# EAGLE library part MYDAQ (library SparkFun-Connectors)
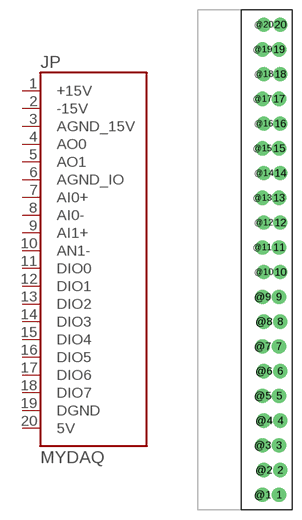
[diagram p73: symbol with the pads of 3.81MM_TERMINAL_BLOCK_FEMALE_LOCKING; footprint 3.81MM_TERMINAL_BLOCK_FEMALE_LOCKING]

Designator prefix JP

## MYDAQ  [3.81MM_TERMINAL_BLOCK_FEMALE_LOCKING]
1  +15V  pwr
2  -15V  pwr
3  AGND_15V  pwr
4  AO0  out
5  AO1  out
6  AGND_IO  pwr
7  AI0+  in
8  AI0-  in
9  AI1+  in
10  AN1-  in
11  DIO0
12  DIO1
13  DIO2
14  DIO3
15  DIO4
16  DIO5
17  DIO6
18  DIO7
19  DGND  pwr
20  5V  pwr

## Footprint 3.81MM_TERMINAL_BLOCK_FEMALE_LOCKING (pad centres in mm)
drill 1.2 pad 2.184: 1 4.521,-36.194; 2 4.724,-32.384; 3 4.521,-28.574; 4 4.724,-24.764; 5 4.521,-20.954; 6 4.724,-17.144; 7 4.521,-13.334; 8 4.724,-9.524; 9 4.521,-5.714; 10 4.724,-1.904; 11 4.521,1.906; 12 4.724,5.716; 13 4.521,9.526; 14 4.724,13.336; 15 4.521,17.146; 16 4.724,20.956; 17 4.521,24.766; 18 4.724,28.576; 19 4.521,32.386; 20 4.724,36.196; @1 1.981,-36.194; @2 2.184,-32.384; @3 1.981,-28.574; @4 2.184,-24.764; @5 1.981,-20.954; @6 2.184,-17.144; @7 1.981,-13.334; @8 2.184,-9.524; @9 1.981,-5.714; @10 2.184,-1.904; @11 1.981,1.906; @12 2.184,5.716; @13 1.981,9.526; @14 2.184,13.336; @15 1.981,17.146; @16 2.184,20.956; @17 1.981,24.766; @18 2.184,28.576; @19 1.981,32.386; @20 2.184,36.196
